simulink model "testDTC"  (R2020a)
settings: Solver=FixedStepDiscrete  StartTime=0.0  StopTime=Inf  FixedStep=Ts  RelTol=1e-3  EnableMultiTasking=on
undefined symbols (not defined in the file or in its folder): A, Compare, conversion, DCAEVT1, DCAEVT1FILT, Digital, Down, Event, Filtered, GPTRIP1SEL, input, Module, of, start, Trip, TZ1, TZ2, Up, version, Zone
libraries: c2802xlib x3

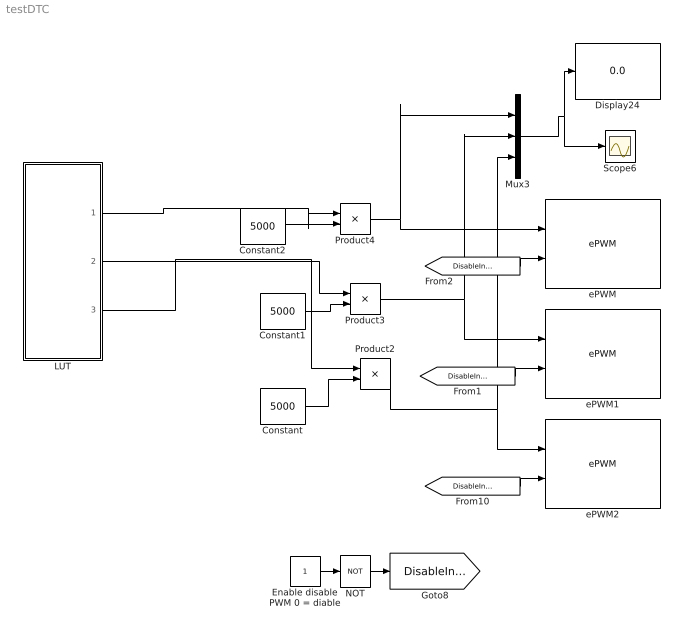
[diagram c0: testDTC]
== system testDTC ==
  Constant : Constant  Value=5000  SampleTime=-1
  Constant1 : Constant  Value=5000  SampleTime=-1
  Constant2 : Constant  Value=5000  SampleTime=-1
  Display24 : Display
  Enable disable PWM 0 = diable : Constant
  LUT : Subsystem
  Mux3 : Mux  Inputs=3
  NOT : Logic  Operator=NOT  IconShape=distinctive  AllPortsSameDT=off  OutDataTypeStr=boolean
  Product2 : Product
  Product3 : Product
  Product4 : Product
  Scope6 : Scope
  ePWM : c2802xlib/ePWM  PwmType=C2000_Type4  useModule=ePWM1  ePWMxLINKTBPRD=Not Linked  periodUnits=Clock cycles  timerSource=Specify via dialog  timerPeriod_clk=5000  timerPeriod_sec=0.0001  tbshadow=Counter equals to zero  countingMode=Up-Down  phaseActiveEnable=Disable  phaseDirection=Count down after sync  phaseActive=0  synchronizationEnable=off  dcaevt1Sync=off  dcbevt1Sync=off  synchronizationOption=Disable  perSynchronizationOption=Counter equals to period (CTR=PRD)  clockPrescale=1  HSclockPrescale=1  enswap=off  ePWMxAStatus=on  ePWMxAactionLogic1=Do nothing  ePWMxAactionLogic2=Do nothing  ePWMxAactionLogic3=Clear  ePWMxAactionLogic4=Set  ePWMxAactionLogic5=Do nothing  ePWMxAactionLogic6=Do nothing  ePWMxACSFenable=off  ePWMxACSFvalue=Forcing disable  ePWMxASFreload=Zero  ePWMxBStatus=on  ePWMxBactionLogic1=Do nothing  ePWMxBactionLogic2=Do nothing  ePWMxBactionLogic3=Set  ePWMxBactionLogic4=Clear  ePWMxBactionLogic5=Do nothing  ePWMxBactionLogic6=Do nothing  ePWMxBCSFenable=off  ePWMxBCSFvalue=Forcing disable  ePWMxBSFreload=Zero  ePWNxBOutWay=off  ePWMxLINKCMPA=Not Linked  CMPAUnits=Clock cycles  CMPASource=Input port  CMPAValue_per=50  CMPAValue_clk=0  enCMPAshadow=Counter equals to zero (CTR=Zero)  ePWMxLINKCMPB=Not Linked  CMPBUnits=Clock cycles  CMPBSource=Specify via dialog  CMPBValue_per=50  CMPBValue_clk=32000  enCMPBshadow=Counter equals to zero (CTR=Zero)  ePWMxLINKCMPC=Not Linked  CMPCUnits=Clock cycles  CMPCSource=Specify via dialog  CMPCValue_per=50  CMPCValue_clk=32000  enCMPCshadow=Counter equals to zero (CTR=Zero)  ePWMxLINKCMPD=Not Linked  CMPDUnits=Clock cycles  CMPDSource=Specify via dialog  CMPDValue_per=50  CMPDValue_clk=32000  enCMPDshadow=Counter equals to zero (CTR=Zero)  enableDBePWMxA=on  enableDBePWMxB=on  enhalfcycle=off  DBpolarity=Active high complementary (AHC)  DBedgeDelay=Positive  DBSource_ePWMxA=ePWMxA  DBSource_ePWMxB=ePWMxA  DBPeriodUnits=Clock cycles  DBperiodSource=Specify via dialog  REDperiod=220  FEDperiod=220  REDperiod_sec=0  FEDperiod_sec=0  LoadModeDBRED=Immediate without using shadow  LoadModeDBFED=Immediate without using shadow  adcstartModuleA=on  adcrequestEventA=First event  adcstartEventA=Digital Compare Module A Event 1 start of conversion (DCAEVT1.soc)  adcstartEventA_type2=Counter equals to period (CTR=PRD)  adcstartModuleB=off  adcrequestEventB=First event  adcstartEventB=Counter equals to zero (CTR=Zero)  adcstartEventB_type2=Counter equals to zero (CTR=Zero)  intEn=off  intPrd=First event  intSel=Counter equals to zero (CTR=Zero)  intSel_type2=Counter equals to zero (CTR=Zero)  hrpe=off  enHRPWM=off  HRPWM_LoadMode=Counter equals to period (CTR=PRD)  HRPWM_CTLMode=Duty or Period control mode  HRPWM_EDGMode=Both edge  hrpeb=off  enHRPWMB=off  HRPWM_LoadModeB=Counter equals to zero (CTR=ZERO)  HRPWM_CTLModeB=Duty or Period control mode  HRPWM_EDGModeB=Both edge  enHRDBRED=off  enHRDBFED=off  enSFO=on  enautoconv=on  chopperEnable=off  chopperFrequency=1  chopperFirstwidth=1  chopperDuty=12.5%  tripZonesource=Input port  tzselOSHT1=off  tzselOSHT2=off  tzselOSHT3=off  tzselOSHDCAEV1=off  tzselOSHDCBEV1=off  tzselCBC1=off  tzselCBC2=off  tzselCBC3=off  tzselCBCDCAEV2=off  tzselCBCDCBEV2=off  tzselOSHT4=off  tzselOSHT5=off  tzselOSHT6=off  tzselCBC4=off  tzselCBC5=off  tzselCBC6=off  enTzOstIntr=off  enTzCbcIntr=off  enTzDCAEVT1Intr=off  enTzDCAEVT2Intr=off  enTzDCBEVT1Intr=off  enTzDCBEVT2Intr=off  ePWMxAforced=Low  ePWMxBforced=Low  DCAEVT1forced=No action  DCBEVT1forced=No action  DCAEVT2forced=No action  DCBEVT2forced=No action  dcah=Trip Zone 1 input (TZ1)  dcal=Trip Zone 2 input (TZ2)  dcbh=Trip Zone 1 input (TZ1)  dcbl=Trip Zone 2 input (TZ2)  dcah_type2=GPTRIP1SEL/(TZ1)  dcal_type2=GPTRIP1SEL/(TZ1)  dcbh_type2=GPTRIP1SEL/(TZ1)  dcbl_type2=GPTRIP1SEL/(TZ1)  gendcaevt1=Event disabled  gendcaevt2=Event disabled  gendcbevt1=Event disabled  gendcbevt2=Event disabled  dcaevt1src=DCAEVT1 with sync  dcaevt2src=DCAEVT2 with sync  dcbevt1src=DCBEVT1 with sync  dcbevt2src=DCBEVT2 with sync  pulsesel=Counter equals to zero (CTR=Zero)  blankinv=off  blankoffset=0  blankwidth=0  evsrcsel=Filtered version of DCAEVT1 (DCAEVT1FILT)  encape=off
  ePWM1 : c2802xlib/ePWM  PwmType=C2000_Type4  useModule=ePWM2  ePWMxLINKTBPRD=Not Linked  periodUnits=Clock cycles  timerSource=Specify via dialog  timerPeriod_clk=5000  timerPeriod_sec=0.0001  tbshadow=Counter equals to zero  countingMode=Up-Down  phaseActiveEnable=Disable  phaseDirection=Count down after sync  phaseActive=0  synchronizationEnable=off  dcaevt1Sync=off  dcbevt1Sync=off  synchronizationOption=Disable  perSynchronizationOption=Counter equals to period (CTR=PRD)  clockPrescale=1  HSclockPrescale=1  enswap=off  ePWMxAStatus=on  ePWMxAactionLogic1=Do nothing  ePWMxAactionLogic2=Do nothing  ePWMxAactionLogic3=Clear  ePWMxAactionLogic4=Set  ePWMxAactionLogic5=Do nothing  ePWMxAactionLogic6=Do nothing  ePWMxACSFenable=off  ePWMxACSFvalue=Forcing disable  ePWMxASFreload=Zero  ePWMxBStatus=on  ePWMxBactionLogic1=Do nothing  ePWMxBactionLogic2=Do nothing  ePWMxBactionLogic3=Set  ePWMxBactionLogic4=Clear  ePWMxBactionLogic5=Do nothing  ePWMxBactionLogic6=Do nothing  ePWMxBCSFenable=off  ePWMxBCSFvalue=Forcing disable  ePWMxBSFreload=Zero  ePWNxBOutWay=off  ePWMxLINKCMPA=Not Linked  CMPAUnits=Clock cycles  CMPASource=Input port  CMPAValue_per=50  CMPAValue_clk=0  enCMPAshadow=Counter equals to zero (CTR=Zero)  ePWMxLINKCMPB=Not Linked  CMPBUnits=Clock cycles  CMPBSource=Specify via dialog  CMPBValue_per=50  CMPBValue_clk=32000  enCMPBshadow=Counter equals to zero (CTR=Zero)  ePWMxLINKCMPC=Not Linked  CMPCUnits=Clock cycles  CMPCSource=Specify via dialog  CMPCValue_per=50  CMPCValue_clk=32000  enCMPCshadow=Counter equals to zero (CTR=Zero)  ePWMxLINKCMPD=Not Linked  CMPDUnits=Clock cycles  CMPDSource=Specify via dialog  CMPDValue_per=50  CMPDValue_clk=32000  enCMPDshadow=Counter equals to zero (CTR=Zero)  enableDBePWMxA=on  enableDBePWMxB=on  enhalfcycle=off  DBpolarity=Active high complementary (AHC)  DBedgeDelay=Positive  DBSource_ePWMxA=ePWMxA  DBSource_ePWMxB=ePWMxA  DBPeriodUnits=Clock cycles  DBperiodSource=Specify via dialog  REDperiod=220  FEDperiod=220  REDperiod_sec=0  FEDperiod_sec=0  LoadModeDBRED=Immediate without using shadow  LoadModeDBFED=Immediate without using shadow  adcstartModuleA=on  adcrequestEventA=First event  adcstartEventA=Digital Compare Module A Event 1 start of conversion (DCAEVT1.soc)  adcstartEventA_type2=Counter equals to period (CTR=PRD)  adcstartModuleB=off  adcrequestEventB=First event  adcstartEventB=Counter equals to zero (CTR=Zero)  adcstartEventB_type2=Counter equals to zero (CTR=Zero)  intEn=off  intPrd=First event  intSel=Counter equals to zero (CTR=Zero)  intSel_type2=Counter equals to zero (CTR=Zero)  hrpe=off  enHRPWM=off  HRPWM_LoadMode=Counter equals to period (CTR=PRD)  HRPWM_CTLMode=Duty or Period control mode  HRPWM_EDGMode=Both edge  hrpeb=off  enHRPWMB=off  HRPWM_LoadModeB=Counter equals to zero (CTR=ZERO)  HRPWM_CTLModeB=Duty or Period control mode  HRPWM_EDGModeB=Both edge  enHRDBRED=off  enHRDBFED=off  enSFO=on  enautoconv=on  chopperEnable=off  chopperFrequency=1  chopperFirstwidth=1  chopperDuty=12.5%  tripZonesource=Input port  tzselOSHT1=off  tzselOSHT2=off  tzselOSHT3=off  tzselOSHDCAEV1=off  tzselOSHDCBEV1=off  tzselCBC1=off  tzselCBC2=off  tzselCBC3=off  tzselCBCDCAEV2=off  tzselCBCDCBEV2=off  tzselOSHT4=off  tzselOSHT5=off  tzselOSHT6=off  tzselCBC4=off  tzselCBC5=off  tzselCBC6=off  enTzOstIntr=off  enTzCbcIntr=off  enTzDCAEVT1Intr=off  enTzDCAEVT2Intr=off  enTzDCBEVT1Intr=off  enTzDCBEVT2Intr=off  ePWMxAforced=Low  ePWMxBforced=Low  DCAEVT1forced=No action  DCBEVT1forced=No action  DCAEVT2forced=No action  DCBEVT2forced=No action  dcah=Trip Zone 1 input (TZ1)  dcal=Trip Zone 2 input (TZ2)  dcbh=Trip Zone 1 input (TZ1)  dcbl=Trip Zone 2 input (TZ2)  dcah_type2=GPTRIP1SEL/(TZ1)  dcal_type2=GPTRIP1SEL/(TZ1)  dcbh_type2=GPTRIP1SEL/(TZ1)  dcbl_type2=GPTRIP1SEL/(TZ1)  gendcaevt1=Event disabled  gendcaevt2=Event disabled  gendcbevt1=Event disabled  gendcbevt2=Event disabled  dcaevt1src=DCAEVT1 with sync  dcaevt2src=DCAEVT2 with sync  dcbevt1src=DCBEVT1 with sync  dcbevt2src=DCBEVT2 with sync  pulsesel=Counter equals to zero (CTR=Zero)  blankinv=off  blankoffset=0  blankwidth=0  evsrcsel=Filtered version of DCAEVT1 (DCAEVT1FILT)  encape=off
  ePWM2 : c2802xlib/ePWM  PwmType=C2000_Type4  useModule=ePWM3  ePWMxLINKTBPRD=Not Linked  periodUnits=Clock cycles  timerSource=Specify via dialog  timerPeriod_clk=5000  timerPeriod_sec=0.0001  tbshadow=Counter equals to zero  countingMode=Up-Down  phaseActiveEnable=Disable  phaseDirection=Count down after sync  phaseActive=0  synchronizationEnable=off  dcaevt1Sync=off  dcbevt1Sync=off  synchronizationOption=Disable  perSynchronizationOption=Counter equals to period (CTR=PRD)  clockPrescale=1  HSclockPrescale=1  enswap=off  ePWMxAStatus=on  ePWMxAactionLogic1=Do nothing  ePWMxAactionLogic2=Do nothing  ePWMxAactionLogic3=Clear  ePWMxAactionLogic4=Set  ePWMxAactionLogic5=Do nothing  ePWMxAactionLogic6=Do nothing  ePWMxACSFenable=off  ePWMxACSFvalue=Forcing disable  ePWMxASFreload=Zero  ePWMxBStatus=on  ePWMxBactionLogic1=Do nothing  ePWMxBactionLogic2=Do nothing  ePWMxBactionLogic3=Set  ePWMxBactionLogic4=Clear  ePWMxBactionLogic5=Do nothing  ePWMxBactionLogic6=Do nothing  ePWMxBCSFenable=off  ePWMxBCSFvalue=Forcing disable  ePWMxBSFreload=Zero  ePWNxBOutWay=off  ePWMxLINKCMPA=Not Linked  CMPAUnits=Clock cycles  CMPASource=Input port  CMPAValue_per=50  CMPAValue_clk=0  enCMPAshadow=Counter equals to zero (CTR=Zero)  ePWMxLINKCMPB=Not Linked  CMPBUnits=Clock cycles  CMPBSource=Specify via dialog  CMPBValue_per=50  CMPBValue_clk=32000  enCMPBshadow=Counter equals to zero (CTR=Zero)  ePWMxLINKCMPC=Not Linked  CMPCUnits=Clock cycles  CMPCSource=Specify via dialog  CMPCValue_per=50  CMPCValue_clk=32000  enCMPCshadow=Counter equals to zero (CTR=Zero)  ePWMxLINKCMPD=Not Linked  CMPDUnits=Clock cycles  CMPDSource=Specify via dialog  CMPDValue_per=50  CMPDValue_clk=32000  enCMPDshadow=Counter equals to zero (CTR=Zero)  enableDBePWMxA=on  enableDBePWMxB=on  enhalfcycle=off  DBpolarity=Active high complementary (AHC)  DBedgeDelay=Positive  DBSource_ePWMxA=ePWMxA  DBSource_ePWMxB=ePWMxA  DBPeriodUnits=Clock cycles  DBperiodSource=Specify via dialog  REDperiod=220  FEDperiod=220  REDperiod_sec=0  FEDperiod_sec=0  LoadModeDBRED=Immediate without using shadow  LoadModeDBFED=Immediate without using shadow  adcstartModuleA=on  adcrequestEventA=First event  adcstartEventA=Digital Compare Module A Event 1 start of conversion (DCAEVT1.soc)  adcstartEventA_type2=Counter equals to period (CTR=PRD)  adcstartModuleB=off  adcrequestEventB=First event  adcstartEventB=Counter equals to zero (CTR=Zero)  adcstartEventB_type2=Counter equals to zero (CTR=Zero)  intEn=off  intPrd=First event  intSel=Counter equals to zero (CTR=Zero)  intSel_type2=Counter equals to zero (CTR=Zero)  hrpe=off  enHRPWM=off  HRPWM_LoadMode=Counter equals to period (CTR=PRD)  HRPWM_CTLMode=Duty or Period control mode  HRPWM_EDGMode=Both edge  hrpeb=off  enHRPWMB=off  HRPWM_LoadModeB=Counter equals to zero (CTR=ZERO)  HRPWM_CTLModeB=Duty or Period control mode  HRPWM_EDGModeB=Both edge  enHRDBRED=off  enHRDBFED=off  enSFO=on  enautoconv=on  chopperEnable=off  chopperFrequency=1  chopperFirstwidth=1  chopperDuty=12.5%  tripZonesource=Input port  tzselOSHT1=off  tzselOSHT2=off  tzselOSHT3=off  tzselOSHDCAEV1=off  tzselOSHDCBEV1=off  tzselCBC1=off  tzselCBC2=off  tzselCBC3=off  tzselCBCDCAEV2=off  tzselCBCDCBEV2=off  tzselOSHT4=off  tzselOSHT5=off  tzselOSHT6=off  tzselCBC4=off  tzselCBC5=off  tzselCBC6=off  enTzOstIntr=off  enTzCbcIntr=off  enTzDCAEVT1Intr=off  enTzDCAEVT2Intr=off  enTzDCBEVT1Intr=off  enTzDCBEVT2Intr=off  ePWMxAforced=Low  ePWMxBforced=Low  DCAEVT1forced=No action  DCBEVT1forced=No action  DCAEVT2forced=No action  DCBEVT2forced=No action  dcah=Trip Zone 1 input (TZ1)  dcal=Trip Zone 2 input (TZ2)  dcbh=Trip Zone 1 input (TZ1)  dcbl=Trip Zone 2 input (TZ2)  dcah_type2=GPTRIP1SEL/(TZ1)  dcal_type2=GPTRIP1SEL/(TZ1)  dcbh_type2=GPTRIP1SEL/(TZ1)  dcbl_type2=GPTRIP1SEL/(TZ1)  gendcaevt1=Event disabled  gendcaevt2=Event disabled  gendcbevt1=Event disabled  gendcbevt2=Event disabled  dcaevt1src=DCAEVT1 with sync  dcaevt2src=DCAEVT2 with sync  dcbevt1src=DCBEVT1 with sync  dcbevt2src=DCBEVT2 with sync  pulsesel=Counter equals to zero (CTR=Zero)  blankinv=off  blankoffset=0  blankwidth=0  evsrcsel=Filtered version of DCAEVT1 (DCAEVT1FILT)  encape=off
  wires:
  LUT/3(Cc) -> Product2/1
  Product2/1 -> Mux3/3, ePWM2/1
  LUT/2(Cb) -> Product3/1
  Constant/1 -> Product2/2
  Product3/1 -> ePWM1/1, Mux3/2
  LUT/1(Ca) -> Product4/1
  [DisableInverter] -> ePWM/2
  Constant2/1 -> Product4/2
  [DisableInverter] -> ePWM1/2
  Product4/1 -> ePWM/1, Mux3/1
  Mux3/1 -> Scope6/1, Display24/1
  Constant1/1 -> Product3/2
  [DisableInverter] -> ePWM2/2
  Enable disable PWM 0 = diable/1 -> NOT/1
  NOT/1 -> [DisableInverter]

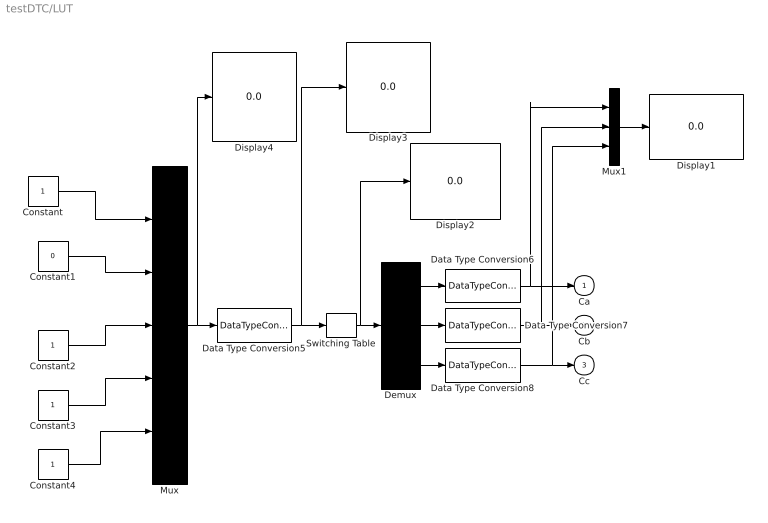
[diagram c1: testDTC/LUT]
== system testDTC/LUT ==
  Constant{,2..4} (4 alike) : Constant
  Constant1 : Constant  Value=0
  Data Type Conversion{5..8} (4 alike) : DataTypeConversion
  Demux : Demux  Outputs=3
  Display{1..4} (4 alike) : Display
  Mux : Mux  Inputs=5
  Mux1 : Mux  Inputs=3
  Switching Table : CombinatorialLogic  TruthTable=Table_2
  Ca : Outport
  Cb : Outport  Port=2
  Cc : Outport  Port=3
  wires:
  Switching Table/1 -> Display2/1, Demux/1
  Data Type Conversion5/1 -> Display3/1, Switching Table/1
  Demux/1 -> Data Type Conversion6/1
  Demux/2 -> Data Type Conversion7/1
  Demux/3 -> Data Type Conversion8/1
  Data Type Conversion6/1 -> Mux1/1, Ca/1
  Data Type Conversion7/1 -> Mux1/2, Cb/1
  Data Type Conversion8/1 -> Mux1/3, Cc/1
  Mux1/1 -> Display1/1
  Mux/1 -> Display4/1, Data Type Conversion5/1
  Constant4/1 -> Mux/5
  Constant3/1 -> Mux/4
  Constant2/1 -> Mux/3
  Constant1/1 -> Mux/2
  Constant/1 -> Mux/1
